| IBIS file stm32h523_533_wlcsp39.ibs
[IBIS ver] 4.2
[File name] stm32h523_533_wlcsp39.ibs
[File Rev] 0.2
[Date] 07-05-2024
[Source] Data Created at STMicroelectronics
[Notes]  File originated from ELDO simulations.
[Disclaimer]  This information is for modeling purpose only and is
   not guaranteed. The information is subject to change without
   notice.
[Copyright] Copyright 2024 STMicroelectronics Inc.
|   Component stm32h523_533_wlcsp39
[Component] stm32h523_533_wlcsp39
[Manufacturer] STMicroelectronics
[Package]
| variable   typ   min   max
R_pkg  0  NA  NA
L_pkg  0  NA  NA
C_pkg  0  NA  NA
[Pin]   signal_name   model_name
A1  PA14  io8_ft_i3c_spi
A3  PA15  io8_ft_i3c_spi
A5  PB3  io8_ft_i3c_spi
A7  PB4  io8_ft_i3c_spi
A9  VCAP  nc
A11  VDD  power
B2  PA12  io8usb_ft_i3c_spi_phy
B4  PA13  io8_ft_i3c_spi
B6  BOOT0  vpphv
B8  VBAT  power
B10  VSS  gnd
C1  PA11  io8usb_ft_i3c_spi_phy
C3  PB7  io8_ft_i3c_spi
C5  PB8  io8_ft_i3c_spi
C7  PC13  io8_ft_i3c_spi_v33
C9  PC15-OSC32_OUT  io_ft_tamp
C11  PC14-OSC32_IN  io_ft_tamp
D2  PA8  io8_ft_i3c_spi
D4  PA3  io8_ft_spi
D6  PA1  io8_ft_spi_tamp
D8  PH1-OSC_OUT  io8_ft_i3c_spi
D10  PH0-OSC_IN  io8_ft_i3c_spi
E1  PB15  io8_ft_spi
E3  PA5  io8_ft_spi
E5  PA4  io8_ft_spi
E7  PA2  io8_ft_spi
E9  PA0  io8_ft_spi
E11  NRST  ioreset_ft_v33
F2  VSS  gnd
F4  PA6  io8_ft_spi
F6  PA7  io8_ft_spi
F8  VSS  gnd
F10  VSSA  nc
G1  VDD  power
G3  VCAP  nc
G5  PB1  io8_ft_spi
G7  PB0  io8_ft_spi
G9  VDD  power
G11  VDDA  nc
[Package Model]   478-wlcsp-39-240122
[Pin Mapping]   pulldown_ref   pullup_ref   | Comment
A1  gndio  vddio
A3  gndio  vddio
A5  gndio  vddio
A7  gndio  vddio
A9  nc  nc
A11  nc  vddio
B2  gndio  vddio
B4  gndio  vddio
B6  gndio  vddio
B8  nc  vsw
B10  gndio  nc
C1  gndio  vddio
C3  gndio  vddio
C5  gndio  vddio
C7  gndio  vddio  | Depending on IO usage
| C7  gndio  vsw  | Depending on IO usage
C9  gndio  vddio  | Depending on IO usage
| C9  gndio  vsw  | Depending on IO usage
C11  gndio  vddio  | Depending on IO usage
| C11  gndio  vsw  | Depending on IO usage
D2  gndio  vddio
D4  gndio  vddio
D6  gndio  vddio
D8  gndio  vddio
D10  gndio  vddio
E1  gndio  vddio
E3  gndio  vddio
E5  gndio  vddio
E7  gndio  vddio
E9  gndio  vddio
E11  gndio  vddio
F2  gndio  nc
F4  gndio  vddio
F6  gndio  vddio
F8  gndio  nc
F10  nc  nc
G1  nc  vddio
G3  nc  nc
G5  gndio  vddio
G7  gndio  vddio
G9  nc  vddio
G11  nc  nc
|[Diff Pin]   inv_pin   vdiff   tdelay_typ   tdelay_min   tdelay_max
|B2   C1   NA   NA   NA   NA
[Model Selector] io8_ft_i3c_spi
io8_ft_spi_ls_1v2 "GPIO SPI - 5V tolerant - low speed - 1.2V range"
io8_ft_spi_ls_1v8 "GPIO SPI - 5V tolerant - low speed - 1.8V range"
io8_ft_spi_ls_3v3 "GPIO SPI - 5V tolerant - low speed - 3.3V range"
io8_ft_spi_ms_1v2 "GPIO SPI - 5V tolerant - med speed - 1.2V range"
io8_ft_spi_ms_1v8 "GPIO SPI - 5V tolerant - med speed - 1.8V range"
io8_ft_spi_ms_3v3 "GPIO SPI - 5V tolerant - med speed - 3.3V range"
io8_ft_spi_fs_1v2 "GPIO SPI - 5V tolerant - fast speed - 1.2V range"
io8_ft_spi_fs_1v8 "GPIO SPI - 5V tolerant - fast speed - 1.8V range"
io8_ft_spi_fs_3v3 "GPIO SPI - 5V tolerant - fast speed - 3.3V range"
io8_ft_spi_hs_1v2 "GPIO SPI - 5V tolerant - high speed - 1.2V range"
io8_ft_spi_hs_1v8 "GPIO SPI - 5V tolerant - high speed - 1.8V range"
io8_ft_spi_hs_3v3 "GPIO SPI - 5V tolerant - high speed - 3.3V range"
io8_ft_hslv_spi_ls_1v2 "GPIO SPI low volt opt - 5V tolerant - low speed - 1.2V range"
io8_ft_hslv_spi_ls_1v8 "GPIO SPI low volt opt - 5V tolerant - low speed - 1.8V range"
io8_ft_hslv_spi_ls_2v5 "GPIO SPI low volt opt - 5V tolerant - low speed - 2.5V range"
io8_ft_hslv_spi_ms_1v2 "GPIO SPI low volt opt - 5V tolerant - med speed - 1.2V range"
io8_ft_hslv_spi_ms_1v8 "GPIO SPI low volt opt - 5V tolerant - med speed - 1.8V range"
io8_ft_hslv_spi_ms_2v5 "GPIO SPI low volt opt - 5V tolerant - med speed - 2.5V range"
io8_ft_hslv_spi_fs_1v2 "GPIO SPI low volt opt - 5V tolerant - fast speed - 1.2V range"
io8_ft_hslv_spi_fs_1v8 "GPIO SPI low volt opt - 5V tolerant - fast speed - 1.8V range"
io8_ft_hslv_spi_fs_2v5 "GPIO SPI low volt opt - 5V tolerant - fast speed - 2.5V range"
io8_ft_hslv_spi_hs_1v2 "GPIO SPI low volt opt - 5V tolerant - high speed - 1.2V range"
io8_ft_hslv_spi_hs_1v8 "GPIO SPI low volt opt - 5V tolerant - high speed - 1.8V range"
io8_ft_hslv_spi_hs_2v5 "GPIO SPI low volt opt - 5V tolerant - high speed - 2.5V range"
io8_ft_i3c_spi_ls_1v2 "GPIO SPI with I3C open-drain - 5V tolerant - low speed - 1.2V range"
io8_ft_i3c_spi_ls_1v8 "GPIO SPI with I3C open-drain - 5V tolerant - low speed - 1.8V range"
io8_ft_i3c_spi_ls_3v3 "GPIO SPI with I3C open-drain - 5V tolerant - low speed - 3.3V range"
io8_ft_i3c_spi_ms_1v2 "GPIO SPI with I3C open-drain - 5V tolerant - med speed - 1.2V range"
io8_ft_i3c_spi_ms_1v8 "GPIO SPI with I3C open-drain - 5V tolerant - med speed - 1.8V range"
io8_ft_i3c_spi_ms_3v3 "GPIO SPI with I3C open-drain - 5V tolerant - med speed - 3.3V range"
io8_ft_i3c_spi_fs_1v2 "GPIO SPI with I3C open-drain - 5V tolerant - fast speed - 1.2V range"
io8_ft_i3c_spi_fs_1v8 "GPIO SPI with I3C open-drain - 5V tolerant - fast speed - 1.8V range"
io8_ft_i3c_spi_fs_3v3 "GPIO SPI with I3C open-drain - 5V tolerant - fast speed - 3.3V range"
io8_ft_i3c_spi_hs_1v2 "GPIO SPI with I3C open-drain - 5V tolerant - high speed - 1.2V range"
io8_ft_i3c_spi_hs_1v8 "GPIO SPI with I3C open-drain - 5V tolerant - high speed - 1.8V range"
io8_ft_i3c_spi_hs_3v3 "GPIO SPI with I3C open-drain - 5V tolerant - high speed - 3.3V range"
io8_ft_hslv_i3c_spi_ls_1v2 "GPIO SPI low volt opt with I3C open-drain - 5V tolerant - low speed - 1.2V range"
io8_ft_hslv_i3c_spi_ls_1v8 "GPIO SPI low volt opt with I3C open-drain - 5V tolerant - low speed - 1.8V range"
io8_ft_hslv_i3c_spi_ls_2v5 "GPIO SPI low volt opt with I3C open-drain - 5V tolerant - low speed - 2.5V range"
io8_ft_hslv_i3c_spi_ms_1v2 "GPIO SPI low volt opt with I3C open-drain - 5V tolerant - med speed - 1.2V range"
io8_ft_hslv_i3c_spi_ms_1v8 "GPIO SPI low volt opt with I3C open-drain - 5V tolerant - med speed - 1.8V range"
io8_ft_hslv_i3c_spi_ms_2v5 "GPIO SPI low volt opt with I3C open-drain - 5V tolerant - med speed - 2.5V range"
io8_ft_hslv_i3c_spi_fs_1v2 "GPIO SPI low volt opt with I3C open-drain - 5V tolerant - fast speed - 1.2V range"
io8_ft_hslv_i3c_spi_fs_1v8 "GPIO SPI low volt opt with I3C open-drain - 5V tolerant - fast speed - 1.8V range"
io8_ft_hslv_i3c_spi_fs_2v5 "GPIO SPI low volt opt with I3C open-drain - 5V tolerant - fast speed - 2.5V range"
io8_ft_hslv_i3c_spi_hs_1v2 "GPIO SPI low volt opt with I3C open-drain - 5V tolerant - high speed - 1.2V range"
io8_ft_hslv_i3c_spi_hs_1v8 "GPIO SPI low volt opt with I3C open-drain - 5V tolerant - high speed - 1.8V range"
io8_ft_hslv_i3c_spi_hs_2v5 "GPIO SPI low volt opt with I3C open-drain - 5V tolerant - high speed - 2.5V range"
io8_ft_i3c_fmp_spi_3v3 "GPIO SPI with I3C fm+ open-drain - 5V tolerant - 3.3V range"
io8_ft_i3c_fmp_spi_1v8 "GPIO SPI with I3C fm+ open-drain - 5V tolerant - 1.8V range"
io8_ft_i3c_fmp_spi_1v2 "GPIO SPI with I3C fm+ open-drain - 5V tolerant - 1.2V range"
[Model Selector] io8_ft_i3c_spi_v33
io8_ft_spi_v33_ls_1v2 ""GPIO SPI V33 - 5V tolerant - low speed - 1.2V range"
io8_ft_spi_v33_ls_1v8 ""GPIO SPI V33 - 5V tolerant - low speed - 1.8V range"
io8_ft_spi_v33_ls_3v3 ""GPIO SPI V33 - 5V tolerant - low speed - 3.3V range"
io8_ft_spi_v33_ms_1v2 ""GPIO SPI V33 - 5V tolerant - med speed - 1.2V range"
io8_ft_spi_v33_ms_1v8 ""GPIO SPI V33 - 5V tolerant - med speed - 1.8V range"
io8_ft_spi_v33_ms_3v3 ""GPIO SPI V33 - 5V tolerant - med speed - 3.3V range"
io8_ft_spi_v33_fs_1v2 ""GPIO SPI V33 - 5V tolerant - fast speed - 1.2V range
io8_ft_spi_v33_fs_1v8 ""GPIO SPI V33 - 5V tolerant - fast speed - 1.8V range
io8_ft_spi_v33_fs_3v3 ""GPIO SPI V33 - 5V tolerant - fast speed - 3.3V range
io8_ft_spi_v33_hs_1v2 ""GPIO SPI V33 - 5V tolerant - high speed - 1.2V range
io8_ft_spi_v33_hs_1v8 ""GPIO SPI V33 - 5V tolerant - high speed - 1.8V range
io8_ft_spi_v33_hs_3v3 ""GPIO SPI V33 - 5V tolerant - high speed - 3.3V range
io8_ft_hslv_spi_v33_ls_1v2 "GPIO SPI V33 low volt opt - 5V tolerant - low speed - 1.2V range""
io8_ft_hslv_spi_v33_ls_1v8 "GPIO SPI V33 low volt opt - 5V tolerant - low speed - 1.8V range""
io8_ft_hslv_spi_v33_ls_2v5 "GPIO SPI V33 low volt opt - 5V tolerant - low speed - 2.5V range""
io8_ft_hslv_spi_v33_ms_1v2 "GPIO SPI V33 low volt opt - 5V tolerant - med speed - 1.2V range""
io8_ft_hslv_spi_v33_ms_1v8 "GPIO SPI V33 low volt opt - 5V tolerant - med speed - 1.8V range""
io8_ft_hslv_spi_v33_ms_2v5 "GPIO SPI V33 low volt opt - 5V tolerant - med speed - 2.5V range""
io8_ft_hslv_spi_v33_fs_1v2 "GPIO SPI V33 low volt opt - 5V tolerant - fast speed - 1.2V range"
io8_ft_hslv_spi_v33_fs_1v8 "GPIO SPI V33 low volt opt - 5V tolerant - fast speed - 1.8V range"
io8_ft_hslv_spi_v33_fs_2v5 "GPIO SPI V33 low volt opt - 5V tolerant - fast speed - 2.5V range"
io8_ft_hslv_spi_v33_hs_1v2 "GPIO SPI V33 low volt opt - 5V tolerant - high speed - 1.2V range"
io8_ft_hslv_spi_v33_hs_1v8 "GPIO SPI V33 low volt opt - 5V tolerant - high speed - 1.8V range"
io8_ft_hslv_spi_v33_hs_2v5 "GPIO SPI V33 low volt opt - 5V tolerant - high speed - 2.5V range"
io8_ft_i3c_spi_v33_ls_1v2 "GPIO SPI V33 with I3C open-drain - 5V tolerant - low speed - 1.2V range"
io8_ft_i3c_spi_v33_ls_1v8 "GPIO SPI V33 with I3C open-drain - 5V tolerant - low speed - 1.8V range"
io8_ft_i3c_spi_v33_ls_3v3 "GPIO SPI V33 with I3C open-drain - 5V tolerant - low speed - 3.3V range"
io8_ft_i3c_spi_v33_ms_1v2 "GPIO SPI V33 with I3C open-drain - 5V tolerant - med speed - 1.2V range"
io8_ft_i3c_spi_v33_ms_1v8 "GPIO SPI V33 with I3C open-drain - 5V tolerant - med speed - 1.8V range"
io8_ft_i3c_spi_v33_ms_3v3 "GPIO SPI V33 with I3C open-drain - 5V tolerant - med speed - 3.3V range"
io8_ft_i3c_spi_v33_fs_1v2 "GPIO SPI V33 with I3C open-drain - 5V tolerant - fast speed - 1.2V range"
io8_ft_i3c_spi_v33_fs_1v8 "GPIO SPI V33 with I3C open-drain - 5V tolerant - fast speed - 1.8V range"
io8_ft_i3c_spi_v33_fs_3v3 "GPIO SPI V33 with I3C open-drain - 5V tolerant - fast speed - 3.3V range"
io8_ft_i3c_spi_v33_hs_1v2 "GPIO SPI V33 with I3C open-drain - 5V tolerant - high speed - 1.2V range"
io8_ft_i3c_spi_v33_hs_1v8 "GPIO SPI V33 with I3C open-drain - 5V tolerant - high speed - 1.8V range"
io8_ft_i3c_spi_v33_hs_3v3 "GPIO SPI V33 with I3C open-drain - 5V tolerant - high speed - 3.3V range"
io8_ft_hslv_i3c_spi_v33_ls_1v2 "GPIO SPI V33 low volt opt with I3C open-drain - 5V tolerant - low speed - 1.2V range"
io8_ft_hslv_i3c_spi_v33_ls_1v8 "GPIO SPI V33 low volt opt with I3C open-drain - 5V tolerant - low speed - 1.8V range"
io8_ft_hslv_i3c_spi_v33_ls_2v5 "GPIO SPI V33 low volt opt with I3C open-drain - 5V tolerant - low speed - 2.5V range"
io8_ft_hslv_i3c_spi_v33_ms_1v2 "GPIO SPI V33 low volt opt with I3C open-drain - 5V tolerant - med speed - 1.2V range"
io8_ft_hslv_i3c_spi_v33_ms_1v8 "GPIO SPI V33 low volt opt with I3C open-drain - 5V tolerant - med speed - 1.8V range"
io8_ft_hslv_i3c_spi_v33_ms_2v5 "GPIO SPI V33 low volt opt with I3C open-drain - 5V tolerant - med speed - 2.5V range"
io8_ft_hslv_i3c_spi_v33_fs_1v2 "GPIO SPI V33 low volt opt with I3C open-drain - 5V tolerant - fast speed - 1.2V range"
io8_ft_hslv_i3c_spi_v33_fs_1v8 "GPIO SPI V33 low volt opt with I3C open-drain - 5V tolerant - fast speed - 1.8V range"
io8_ft_hslv_i3c_spi_v33_fs_2v5 "GPIO SPI V33 low volt opt with I3C open-drain - 5V tolerant - fast speed - 2.5V range"
io8_ft_hslv_i3c_spi_v33_hs_1v2 "GPIO SPI V33 low volt opt with I3C open-drain - 5V tolerant - high speed - 1.2V range"
io8_ft_hslv_i3c_spi_v33_hs_1v8 "GPIO SPI V33 low volt opt with I3C open-drain - 5V tolerant - high speed - 1.8V range"
io8_ft_hslv_i3c_spi_v33_hs_2v5 "GPIO SPI V33 low volt opt with I3C open-drain - 5V tolerant - high speed - 2.5V range"
io8_ft_i3c_fmp_spi_v33_3v3 "GPIO SPI V33 with I3C fm+ open-drain - 5V tolerant - 3.3V range"
io8_ft_i3c_fmp_spi_v33_1v8 "GPIO SPI V33 with I3C fm+ open-drain - 5V tolerant - 1.8V range"
io8_ft_i3c_fmp_spi_v33_1v2 "GPIO SPI V33 with I3C fm+ open-drain - 5V tolerant - 1.2V range"
[Model Selector] io8_ft_spi
io8_ft_spi_ls_1v2 "GPIO SPI - 5V tolerant - low speed - 1.2V range"
io8_ft_spi_ls_1v8 "GPIO SPI - 5V tolerant - low speed - 1.8V range"
io8_ft_spi_ls_3v3 "GPIO SPI - 5V tolerant - low speed - 3.3V range"
io8_ft_spi_ms_1v2 "GPIO SPI- 5V tolerant - med speed - 1.2V range"
io8_ft_spi_ms_1v8 "GPIO SPI- 5V tolerant - med speed - 1.8V range"
io8_ft_spi_ms_3v3 "GPIO SPI- 5V tolerant - med speed - 3.3V range"
io8_ft_spi_fs_1v2 "GPIO SPI- 5V tolerant - fast speed - 1.2V range"
io8_ft_spi_fs_1v8 "GPIO SPI- 5V tolerant - fast speed - 1.8V range"
io8_ft_spi_fs_3v3 "GPIO SPI- 5V tolerant - fast speed - 3.3V range"
io8_ft_spi_hs_1v2 "GPIO SPI- 5V tolerant - high speed - 1.2V range"
io8_ft_spi_hs_1v8 "GPIO SPI- 5V tolerant - high speed - 1.8V range"
io8_ft_spi_hs_3v3 "GPIO SPI- 5V tolerant - high speed - 3.3V range"
io8_ft_hslv_spi_ls_1v2 "GPIO SPI low volt opt - 5V tolerant - low speed - 1.2V range"
io8_ft_hslv_spi_ls_1v8 "GPIO SPI low volt opt - 5V tolerant - low speed - 1.8V range"
io8_ft_hslv_spi_ls_2v5 "GPIO SPI low volt opt - 5V tolerant - low speed - 2.5V range"
io8_ft_hslv_spi_ms_1v2 "GPIO SPI low volt opt - 5V tolerant - med speed - 1.2V range"
io8_ft_hslv_spi_ms_1v8 "GPIO SPI low volt opt - 5V tolerant - med speed - 1.8V range"
io8_ft_hslv_spi_ms_2v5 "GPIO SPI low volt opt - 5V tolerant - med speed - 2.5V range"
io8_ft_hslv_spi_fs_1v2 "GPIO SPI low volt opt - 5V tolerant - fast speed - 1.2V range"
io8_ft_hslv_spi_fs_1v8 "GPIO SPI low volt opt - 5V tolerant - fast speed - 1.8V range"
io8_ft_hslv_spi_fs_2v5 "GPIO SPI low volt opt - 5V tolerant - fast speed - 2.5V range"
io8_ft_hslv_spi_hs_1v2 "GPIO SPI low volt opt - 5V tolerant - high speed - 1.2V range"
io8_ft_hslv_spi_hs_1v8 "GPIO SPI low volt opt - 5V tolerant - high speed - 1.8V range"
io8_ft_hslv_spi_hs_2v5 "GPIO SPI low volt opt - 5V tolerant - high speed - 2.5V range"
[Model Selector] io8_ft_spi_tamp
io8_ft_spi_ls_1v2 "GPIO SPI - 5V tolerant - low speed - 1.2V range"
io8_ft_spi_ls_1v8 "GPIO SPI - 5V tolerant - low speed - 1.8V range"
io8_ft_spi_ls_3v3 "GPIO SPI- 5V tolerant - low speed - 3.3V range"
io8_ft_spi_ms_1v2 "GPIO SPI - 5V tolerant - med speed - 1.2V range"
io8_ft_spi_ms_1v8 "GPIO SPI - 5V tolerant - med speed - 1.8V range"
io8_ft_spi_ms_3v3 "GPIO SPI - 5V tolerant - med speed - 3.3V range"
io8_ft_spi_fs_1v2 "GPIO SPI - 5V tolerant - fast speed - 1.2V range"
io8_ft_spi_fs_1v8 "GPIO SPI - 5V tolerant - fast speed - 1.8V range"
io8_ft_spi_fs_3v3 "GPIO SPI - 5V tolerant - fast speed - 3.3V range"
io8_ft_spi_hs_1v2 "GPIO SPI - 5V tolerant - high speed - 1.2V range"
io8_ft_spi_hs_1v8 "GPIO SPI - 5V tolerant - high speed - 1.8V range"
io8_ft_spi_hs_3v3 "GPIO SPI - 5V tolerant - high speed - 3.3V range"
io8_ft_hslv_spi_ls_1v2 "GPIO SPI low volt opt - 5V tolerant - low speed - 1.2V range"
io8_ft_hslv_spi_ls_1v8 "GPIO SPI low volt opt - 5V tolerant - low speed - 1.8V range"
io8_ft_hslv_spi_ls_2v5 "GPIO SPI low volt opt - 5V tolerant - low speed - 2.5V range"
io8_ft_hslv_spi_ms_1v2 "GPIO SPI low volt opt - 5V tolerant - med speed - 1.2V range"
io8_ft_hslv_spi_ms_1v8 "GPIO SPI low volt opt - 5V tolerant - med speed - 1.8V range"
io8_ft_hslv_spi_ms_2v5 "GPIO SPI low volt opt - 5V tolerant - med speed - 2.5V range"
io8_ft_hslv_spi_fs_1v2 "GPIO SPI low volt opt - 5V tolerant - fast speed - 1.2V range"
io8_ft_hslv_spi_fs_1v8 "GPIO SPI low volt opt - 5V tolerant - fast speed - 1.8V range"
io8_ft_hslv_spi_fs_2v5 "GPIO SPI low volt opt - 5V tolerant - fast speed - 2.5V range"
io8_ft_hslv_spi_hs_1v2 "GPIO SPI low volt opt - 5V tolerant - high speed - 1.2V range"
io8_ft_hslv_spi_hs_1v8 "GPIO SPI low volt opt - 5V tolerant - high speed - 1.8V range"
io8_ft_hslv_spi_hs_2v5 "GPIO SPI low volt opt - 5V tolerant - high speed - 2.5V range
io8_ft_tamp_v33_1v2 "IO tamper - 5V tolerant - 1.2V range"
io8_ft_tamp_v33_1v8 "IO tamper - 5V tolerant - 1.8V range"
io8_ft_tamp_v33_3v3 "IO tamper - 5V tolerant - 3.3V range"
[Model Selector] io8usb_ft_i3c_spi_phy
io8_ft_spi_ls_1v2 "GPIO SPI - 5V tolerant - low speed - 1.2V range"
io8_ft_spi_ls_1v8 "GPIO SPI - 5V tolerant - low speed - 1.8V range"
io8_ft_spi_ls_3v3 "GPIO SPI - 5V tolerant - low speed - 3.3V range"
io8_ft_spi_ms_1v2 "GPIO SPI - 5V tolerant - med speed - 1.2V range"
io8_ft_spi_ms_1v8 "GPIO SPI - 5V tolerant - med speed - 1.8V range"
io8_ft_spi_ms_3v3 "GPIO SPI - 5V tolerant - med speed - 3.3V range"
io8_ft_spi_fs_1v2 "GPIO SPI - 5V tolerant - fast speed - 1.2V range"
io8_ft_spi_fs_1v8 "GPIO SPI - 5V tolerant - fast speed - 1.8V range"
io8_ft_spi_fs_3v3 "GPIO SPI - 5V tolerant - fast speed - 3.3V range"
io8_ft_spi_hs_1v2 "GPIO SPI - 5V tolerant - high speed - 1.2V range"
io8_ft_spi_hs_1v8 "GPIO SPI - 5V tolerant - high speed - 1.8V range"
io8_ft_spi_hs_3v3 "GPIO SPI - 5V tolerant - high speed - 3.3V range"
io8_ft_hslv_spi_ls_1v2 "GPIO SPI low volt opt - 5V tolerant - low speed - 1.2V range"
io8_ft_hslv_spi_ls_1v8 "GPIO SPI low volt opt - 5V tolerant - low speed - 1.8V range"
io8_ft_hslv_spi_ls_2v5 "GPIO SPI low volt opt - 5V tolerant - low speed - 2.5V range"
io8_ft_hslv_spi_ms_1v2 "GPIO SPI low volt opt - 5V tolerant - med speed - 1.2V range"
io8_ft_hslv_spi_ms_1v8 "GPIO SPI low volt opt - 5V tolerant - med speed - 1.8V range"
io8_ft_hslv_spi_ms_2v5 "GPIO SPI low volt opt - 5V tolerant - med speed - 2.5V range"
io8_ft_hslv_spi_fs_1v2 "GPIO SPI low volt opt - 5V tolerant - fast speed - 1.2V range"
io8_ft_hslv_spi_fs_1v8 "GPIO SPI low volt opt - 5V tolerant - fast speed - 1.8V range"
io8_ft_hslv_spi_fs_2v5 "GPIO SPI low volt opt - 5V tolerant - fast speed - 2.5V range"
io8_ft_hslv_spi_hs_1v2 "GPIO SPI low volt opt - 5V tolerant - high speed - 1.2V range"
io8_ft_hslv_spi_hs_1v8 "GPIO SPI low volt opt - 5V tolerant - high speed - 1.8V range"
io8_ft_hslv_spi_hs_2v5 "GPIO SPI low volt opt - 5V tolerant - high speed - 2.5V range"
io8_ft_i3c_spi_ls_1v2 "GPIO SPI  with I3C open-drain - 5V tolerant - low speed - 1.2V range"
io8_ft_i3c_spi_ls_1v8 "GPIO SPI  with I3C open-drain - 5V tolerant - low speed - 1.8V range"
io8_ft_i3c_spi_ls_3v3 "GPIO SPI  with I3C open-drain - 5V tolerant - low speed - 3.3V range"
io8_ft_i3c_spi_ms_1v2 "GPIO SPI  with I3C open-drain - 5V tolerant - med speed - 1.2V range"
io8_ft_i3c_spi_ms_1v8 "GPIO SPI  with I3C open-drain - 5V tolerant - med speed - 1.8V range"
io8_ft_i3c_spi_ms_3v3 "GPIO SPI  with I3C open-drain - 5V tolerant - med speed - 3.3V range"
io8_ft_i3c_spi_fs_1v2 "GPIO SPI  with I3C open-drain - 5V tolerant - fast speed - 1.2V range"
io8_ft_i3c_spi_fs_1v8 "GPIO SPI  with I3C open-drain - 5V tolerant - fast speed - 1.8V range"
io8_ft_i3c_spi_fs_3v3 "GPIO SPI  with I3C open-drain - 5V tolerant - fast speed - 3.3V range"
io8_ft_i3c_spi_hs_1v2 "GPIO SPI  with I3C open-drain - 5V tolerant - high speed - 1.2V range"
io8_ft_i3c_spi_hs_1v8 "GPIO SPI  with I3C open-drain - 5V tolerant - high speed - 1.8V range"
io8_ft_i3c_spi_hs_3v3 "GPIO SPI  with I3C open-drain - 5V tolerant - high speed - 3.3V range"
io8_ft_hslv_i3c_spi_ls_1v2 "GPIO SPI  low volt opt with I3C open-drain - 5V tolerant - low speed - 1.2V range"
io8_ft_hslv_i3c_spi_ls_1v8 "GPIO SPI  low volt opt with I3C open-drain - 5V tolerant - low speed - 1.8V range"
io8_ft_hslv_i3c_spi_ls_2v5 "GPIO SPI  low volt opt with I3C open-drain - 5V tolerant - low speed - 2.5V range"
io8_ft_hslv_i3c_spi_ms_1v2 "GPIO SPI  low volt opt with I3C open-drain - 5V tolerant - med speed - 1.2V range"
io8_ft_hslv_i3c_spi_ms_1v8 "GPIO SPI  low volt opt with I3C open-drain - 5V tolerant - med speed - 1.8V range"
io8_ft_hslv_i3c_spi_ms_2v5 "GPIO SPI  low volt opt with I3C open-drain - 5V tolerant - med speed - 2.5V range"
io8_ft_hslv_i3c_spi_fs_1v2 "GPIO SPI  low volt opt with I3C open-drain - 5V tolerant - fast speed - 1.2V range"
io8_ft_hslv_i3c_spi_fs_1v8 "GPIO SPI  low volt opt with I3C open-drain - 5V tolerant - fast speed - 1.8V range"
io8_ft_hslv_i3c_spi_fs_2v5 "GPIO SPI  low volt opt with I3C open-drain - 5V tolerant - fast speed - 2.5V range"
io8_ft_hslv_i3c_spi_hs_1v2 "GPIO SPI  low volt opt with I3C open-drain - 5V tolerant - high speed - 1.2V range"
io8_ft_hslv_i3c_spi_hs_1v8 "GPIO SPI  low volt opt with I3C open-drain - 5V tolerant - high speed - 1.8V range"
io8_ft_hslv_i3c_spi_hs_2v5 "GPIO SPI  low volt opt with I3C open-drain - 5V tolerant - high speed - 2.5V range"
io8_ft_i3c_fmp_spi_3v3 "GPIO SPI  with I3C fm+ open-drain - 5V tolerant - 3.3V range"
io8_ft_i3c_fmp_spi_1v8 "GPIO SPI  with I3C fm+ open-drain - 5V tolerant - 1.8V range"
io8_ft_i3c_fmp_spi_1v2 "GPIO SPI  with I3C fm+ open-drain - 5V tolerant - 1.2V range"
io8usb_ft_phy_ls_2v5 "USB PHY - 5V tolerant - low speed - 2.5V range"
io8usb_ft_phy_ls_3v3 "USB PHY - 5V tolerant - low speed - 3.3V range
io8usb_ft_phy_fs_2v5 "USB PHY - 5V tolerant - fast speed - 2.5V range"
io8usb_ft_phy_fs_3v3 "USB PHY - 5V tolerant - fast speed - 3.3V range"
[Model Selector] io_ft_tamp
io_ft_tamp_3v3 "IO tamper - 5V tolerant - 3.3V range"
io_ft_tamp_1v8 "IO tamper - 5V tolerant - 1.8V range"
io_ft_tamp_1v2 "IO tamper - 5V tolerant - 1.2V range"
[Model Selector] ioreset_ft_v33
ioreset_ft_v33_1v2 "Reset PAD. 5V tolerant. 1.2V range"
ioreset_ft_v33_1v8 "Reset PAD. 5V tolerant. 1.8V range"
ioreset_ft_v33_3v3 "Reset PAD. 5V tolerant. 3.3V range"
[Model Selector] vpphv
vpphv_1v2 "Flash Test cell v33 = 1.2 V range"
vpphv_1v8 "Flash Test cell v33 = 1.8 V range"
vpphv_3v3 "Flash Test cell v33 = 3.3 V range"
[Define Package Model]  478-wlcsp-39-240122
[Manufacturer]  Unknown
[OEM]  Unknown
[Description]  None
[Number Of Pins]  35
[Pin Numbers]
| Pin Num   Terminal Name
B6 | BOOT0
E11 | NRST
E9 | PA0
D6 | PA1
E7 | PA2
D4 | PA3
E5 | PA4
E3 | PA5
F4 | PA6
F6 | PA7
D2 | PA8
C1 | PA11
B2 | PA12
B4 | PA13
A1 | PA14
A3 | PA15
G7 | PB0
G5 | PB1
A5 | PB3
A7 | PB4
C3 | PB7
C5 | PB8
E1 | PB15
C7 | PC13
C11 | PC14-OSC32_IN
C9 | PC15-OSC32_OUT
D10 | PH0-OSC_IN
D8 | PH1-OSC_OUT
B8 | VBAT
G3 | VCAP
A9 | VCAP
A11 | VDD
G11 | VDDA
B10 | VSS
F10 | VSSA
|[Merged Pins]  A11
|G1  |  VDD
|G9  |  VDD
|[Merged Pins]  B10
|F2  |  VSS
|F8  |  VSS
[Model Data]
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[End Model Data]
[End Package Model]
|End [Component]
| Models and submodels in the file (118): io8_ft_hslv_i3c_spi_fs_1v2 (I/O_open_drain), io8_ft_hslv_i3c_spi_fs_1v8 (I/O_open_drain), io8_ft_hslv_i3c_spi_fs_2v5 (I/O_open_drain), io8_ft_hslv_i3c_spi_hs_1v2 (I/O_open_drain), io8_ft_hslv_i3c_spi_hs_1v8 (I/O_open_drain), io8_ft_hslv_i3c_spi_hs_2v5 (I/O_open_drain), io8_ft_hslv_i3c_spi_ls_1v2 (I/O_open_drain), io8_ft_hslv_i3c_spi_ls_1v8 (I/O_open_drain), io8_ft_hslv_i3c_spi_ls_2v5 (I/O_open_drain), io8_ft_hslv_i3c_spi_ms_1v2 (I/O_open_drain), io8_ft_hslv_i3c_spi_ms_1v8 (I/O_open_drain), io8_ft_hslv_i3c_spi_ms_2v5 (I/O_open_drain), io8_ft_hslv_i3c_spi_v33_fs_1v2 (I/O_open_drain), io8_ft_hslv_i3c_spi_v33_fs_1v8 (I/O_open_drain), io8_ft_hslv_i3c_spi_v33_fs_2v5 (I/O_open_drain), io8_ft_hslv_i3c_spi_v33_hs_1v2 (I/O_open_drain), io8_ft_hslv_i3c_spi_v33_hs_1v8 (I/O_open_drain), io8_ft_hslv_i3c_spi_v33_hs_2v5 (I/O_open_drain), io8_ft_hslv_i3c_spi_v33_ls_1v2 (I/O_open_drain), io8_ft_hslv_i3c_spi_v33_ls_1v8 (I/O_open_drain), io8_ft_hslv_i3c_spi_v33_ls_2v5 (I/O_open_drain), io8_ft_hslv_i3c_spi_v33_ms_1v2 (I/O_open_drain), io8_ft_hslv_i3c_spi_v33_ms_1v8 (I/O_open_drain), io8_ft_hslv_i3c_spi_v33_ms_2v5 (I/O_open_drain), io8_ft_hslv_spi_fs_1v2 (I/O), io8_ft_hslv_spi_fs_1v8 (I/O), io8_ft_hslv_spi_fs_2v5 (I/O), io8_ft_hslv_spi_hs_1v2 (I/O), io8_ft_hslv_spi_hs_1v8 (I/O), io8_ft_hslv_spi_hs_2v5 (I/O), io8_ft_hslv_spi_ls_1v2 (I/O), io8_ft_hslv_spi_ls_1v8 (I/O), io8_ft_hslv_spi_ls_2v5 (I/O), io8_ft_hslv_spi_ms_1v2 (I/O), io8_ft_hslv_spi_ms_1v8 (I/O), io8_ft_hslv_spi_ms_2v5 (I/O), io8_ft_hslv_spi_v33_fs_1v2 (I/O), io8_ft_hslv_spi_v33_fs_1v8 (I/O), io8_ft_hslv_spi_v33_fs_2v5 (I/O), io8_ft_hslv_spi_v33_hs_1v2 (I/O), io8_ft_hslv_spi_v33_hs_1v8 (I/O), io8_ft_hslv_spi_v33_hs_2v5 (I/O), io8_ft_hslv_spi_v33_ls_1v2 (I/O), io8_ft_hslv_spi_v33_ls_1v8 (I/O), io8_ft_hslv_spi_v33_ls_2v5 (I/O), io8_ft_hslv_spi_v33_ms_1v2 (I/O), io8_ft_hslv_spi_v33_ms_1v8 (I/O), io8_ft_hslv_spi_v33_ms_2v5 (I/O), io8_ft_i3c_fmp_spi_1v2 (I/O_open_drain), io8_ft_i3c_fmp_spi_1v8 (I/O_open_drain), io8_ft_i3c_fmp_spi_3v3 (I/O_open_drain), io8_ft_i3c_fmp_spi_v33_1v2 (I/O_open_drain), io8_ft_i3c_fmp_spi_v33_1v8 (I/O_open_drain), io8_ft_i3c_fmp_spi_v33_3v3 (I/O_open_drain), io8_ft_i3c_spi_fs_1v2 (I/O_open_drain), io8_ft_i3c_spi_fs_1v8 (I/O_open_drain), io8_ft_i3c_spi_fs_3v3 (I/O_open_drain), io8_ft_i3c_spi_hs_1v2 (I/O_open_drain), io8_ft_i3c_spi_hs_1v8 (I/O_open_drain), io8_ft_i3c_spi_hs_3v3 (I/O_open_drain), io8_ft_i3c_spi_ls_1v2 (I/O_open_drain), io8_ft_i3c_spi_ls_1v8 (I/O_open_drain), io8_ft_i3c_spi_ls_3v3 (I/O_open_drain), io8_ft_i3c_spi_ms_1v2 (I/O_open_drain), io8_ft_i3c_spi_ms_1v8 (I/O_open_drain), io8_ft_i3c_spi_ms_3v3 (I/O_open_drain), io8_ft_i3c_spi_v33_fs_1v2 (I/O_open_drain), io8_ft_i3c_spi_v33_fs_1v8 (I/O_open_drain), io8_ft_i3c_spi_v33_fs_3v3 (I/O_open_drain), io8_ft_i3c_spi_v33_hs_1v2 (I/O_open_drain), io8_ft_i3c_spi_v33_hs_1v8 (I/O_open_drain), io8_ft_i3c_spi_v33_hs_3v3 (I/O_open_drain), io8_ft_i3c_spi_v33_ls_1v2 (I/O_open_drain), io8_ft_i3c_spi_v33_ls_1v8 (I/O_open_drain), io8_ft_i3c_spi_v33_ls_3v3 (I/O_open_drain), io8_ft_i3c_spi_v33_ms_1v2 (I/O_open_drain), io8_ft_i3c_spi_v33_ms_1v8 (I/O_open_drain), io8_ft_i3c_spi_v33_ms_3v3 (I/O_open_drain), io8_ft_spi_fs_1v2 (I/O), io8_ft_spi_fs_1v8 (I/O)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
